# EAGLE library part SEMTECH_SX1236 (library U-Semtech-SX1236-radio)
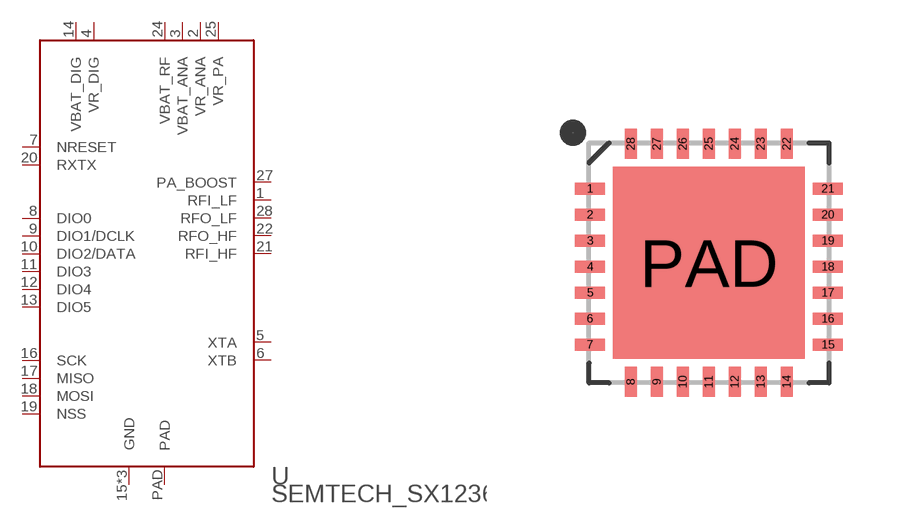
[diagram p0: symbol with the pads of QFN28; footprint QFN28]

Designator prefix U

## SEMTECH_SX1236  [QFN28]
1  RFI_LF
2  VR_ANA  pwr
3  VBAT_ANA  pwr
4  VR_DIG  pwr
5  XTA
6  XTB
7  NRESET  in
8  DIO0
9  DIO1/DCLK
10  DIO2/DATA
11  DIO3
12  DIO4
13  DIO5
14  VBAT_DIG  pwr
15  GND  pwr
16  SCK  in
17  MISO  out
18  MOSI  in
19  NSS  in
20  RXTX  out
21  RFI_HF
22  RFO_HF
23  GND  pwr
24  VBAT_RF  pwr
25  VR_PA  pwr
26  GND  pwr
27  PA_BOOST
28  RFO_LF
PAD  PAD  pwr

## Footprint QFN28 (pad centres in mm)
smd 0.75 x 0.3: 1 -2.975,1.95; 2 -2.975,1.3; 3 -2.975,0.65; 4 -2.975,0; 5 -2.975,-0.65; 6 -2.975,-1.3; 7 -2.975,-1.95; 15 2.975,-1.95; 16 2.975,-1.3; 17 2.975,-0.65; 18 2.975,0; 19 2.975,0.65; 20 2.975,1.3; 21 2.975,1.95
smd 0.3 x 0.75: 8 -1.95,-2.875; 9 -1.3,-2.875; 10 -0.65,-2.875; 11 0,-2.875; 12 0.65,-2.875; 13 1.3,-2.875; 14 1.95,-2.875; 22 1.95,3.075; 23 1.3,3.075; 24 0.65,3.075; 25 0,3.075; 26 -0.65,3.075; 27 -1.3,3.075; 28 -1.95,3.075
smd 4.8 x 4.8: PAD 0,0.1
